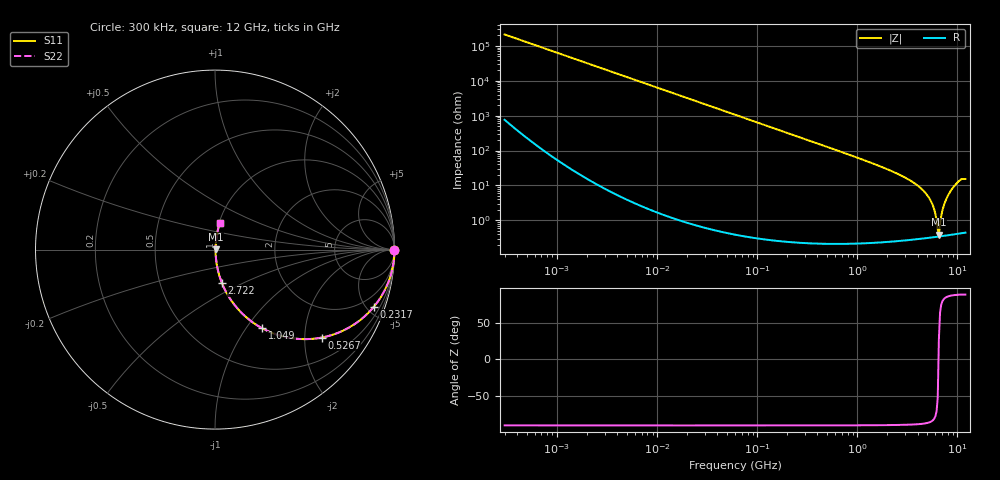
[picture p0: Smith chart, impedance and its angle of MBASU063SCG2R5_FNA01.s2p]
! MBASU063SCG2R5_FNA01  S-PARAMETER MODEL  ( General Type )
! Model Generated by TAIYO YUDEN Corporation (http://www.ty-top.com)
! Version 1.0
! TAIYO YUDEN Control No. 130801
! Copyright(c) 2013 TAIYO YUDEN CO.,LTD. All Rights Reserved.
! Product Description (link to TY-COMPAS)
! https://ds.yuden.co.jp/TYCOMPAS/or/detail?pn=MBASU063SCG2R5CFNA01&u=M
! Products Name : Multilayer Ceramic Capacitors
! Characteristics :
!  Capacitance : 2.5 pF , Rated Voltage : 50V , TCC : CG / C0G
!  Case Size : 0.6 x 0.3 / 0.024 x 0.012 [mm/inch] , Thickness : 0.3 / 0.012 [mm/inch]
!  (Conditions: Temperature = 25 degC , DC Bias Current/Voltage = 0A / 0V)
! External Node Assignments :
!  1  o---| |---o  2
! GND o---------o GND
! Frequency Range : 0.3MHz  -  12000MHz  [ 401 STEP ]
# MHz S RI R 50
! Freq[MHz].  S11 Real  S11 Imag  S21 Real  S21 Imag  S12 Real  S12 Imag  S22 Real  S22 Imag
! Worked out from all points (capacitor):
!   401 points, 300 kHz to 12 GHz, reference 50 ohm
!   read as one part in series: C = 2.48 pF near 316.3 kHz
!   lowest |Z| = 389 mohm at 6.525 GHz (marker M1)
!   series resonance near 6.474 GHz, so ESL is about 240 pH
!   S11 on the Smith chart (normalised r, x): 300 kHz: open; 231.7 MHz: 1.00, -5.53; 526.7 MHz: 1.00, -2.42; 1.049 GHz: 1.00, -1.19; 2.722 GHz: 1.01, -0.39; 12 GHz: 1.01, +0.31
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0.3  1 -0.000468  1.88e-06 0.000468  1.88e-06 0.000468  1 -0.000468
1.769972  1 -0.00276  9.05e-06 0.00276  9.05e-06 0.00276  1 -0.00276
10.44266  0.9997 -0.0163  0.000269 0.0163  0.000269 0.0163  0.9997 -0.0163
60  0.9913 -0.0927  0.0087 0.0927  0.0087 0.0927  0.9913 -0.0927
231.6935  0.8842 -0.3196  0.1158 0.3196  0.1158 0.3196  0.8842 -0.3196
353.9943  0.7653 -0.4232  0.2347 0.4232  0.2347 0.4232  0.7653 -0.4232
526.7124  0.594 -0.4902  0.406 0.4902  0.406 0.4902  0.594 -0.4902
1048.836  0.2627 -0.4383  0.7373 0.4383  0.7373 0.4383  0.2627 -0.4383
2088.533  0.0724 -0.2548  0.9276 0.2548  0.9276 0.2548  0.0724 -0.2548
2722.03  0.0387 -0.1863  0.9613 0.1863  0.9613 0.1863  0.0387 -0.1863
3841.137  0.0144 -0.1067  0.9856 0.1067  0.9856 0.1067  0.0144 -0.1067
4875.354  0.00632 -0.0568  0.9937 0.0568  0.9937 0.0568  0.00632 -0.0568
5565.855  0.00414 -0.0303  0.9959 0.0303  0.9959 0.0303  0.00414 -0.0303
5868.704  0.00368 -0.0198  0.9963 0.0198  0.9963 0.0198  0.00368 -0.0198
6188.031  0.00344 -0.0094  0.9966 0.0094  0.9966 0.0094  0.00344 -0.0094
6354.153  0.0034 -0.00427  0.9966 0.00427  0.9966 0.00427  0.0034 -0.00427
6524.734  0.00342 0.00182  0.9966 -0.00182  0.9966 -0.00182  0.00342 0.00182
6699.894  0.0035 0.00694  0.9965 -0.00694  0.9965 -0.00694  0.0035 0.00694
7448.838  0.00455 0.0308  0.9954 -0.0308  0.9954 -0.0308  0.00455 0.0308
8281.503  0.00728 0.0591  0.9927 -0.0591  0.9927 -0.0591  0.00728 0.0591
10236.47  0.0205 0.1268  0.9795 -0.1268  0.9795 -0.1268  0.0205 0.1268
12000  0.0269 0.1481  0.9731 -0.1481  0.9731 -0.1481  0.0269 0.1481
